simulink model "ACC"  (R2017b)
settings: Solver=FixedStepDiscrete  StartTime=0.0  StopTime=10.0  FixedStep=0.01  RelTol=1e-3  EnableMultiTasking=on
undefined symbols (not defined in the file): ACC_CONST0_NUMB, ACC_CONST1000_NUMB, ACC_CONST100_NUMB, ACC_CONST121_NUMB, ACC_CONST1_NUMB, ACC_CONST2047_NUMB, ACC_CONST60000_NUMB, ACC_CONST60_NUMB, ACC_CONSTF1_NUMB, ACC_RUNTIME_MS, ASWTYPE_FALSE, ASWTYPE_TRUE, CcACC_ACChrgDispSOCPrmt_pct, CcACC_ACChrgMismatch_ms, CcACC_ACChrgPACKVolLim_V, CcACC_ACChrgPACKVolLimTi_ms, CcACC_ACChrgPrmtObcFltLvl_numb, CcACC_ACChrgPrmtVcuFltLvl_numb, CcACC_ACChrgStepCurr_A, CcACC_ACChrgTempPrmtDelayTime_ms, CcACC_ACCrntUnctrolTi_ms, CcACC_ACFullChrgHysVolt_mV, CcACC_ACFullStepChrgTi1_ms, CcACC_ACFullStepChrgTi2_ms, CcACC_ACMaxChrgCurr_A, CcACC_ACStepChrgWaitTime_ms, CcACC_ACStop2DefaultTi_ms, CcACC_ACStop2DefaultTiDelay_ms, CcACC_BatFullResetTime_ms, CcACC_ChrgCrnt0HysVolt_mV, CcACC_ChrgEndDeviationVol1_mV, CcACC_ChrgEndDeviationVol2_mV, CcACC_ChrgEndDeviationVol3_mV, CcACC_ChrgMaxPackVoltLimt_V, CcACC_ChrgPwr1_W, CcACC_ChrgPwr2_W, CcACC_ChrgPwr3_W, CcACC_ChrgSt2StepChrgDeviVol_mV, CcACC_ChrgSt2StepChrgTime_ms, CcACC_ChrgStCutoffTime_ms, CcACC_ChrgStFullChrgCrnt_A, CcACC_CPDutyLowThrhd_pct, CcACC_CrntFilterTi1_cnt, CcACC_CrntFilterTi2_cnt, CcACC_CrntFilterTi2_ms, CcACC_CurrObcPreHeatLowThrhd_A, CcACC_DiffACChrgCrnt_A, CcACC_DiffACChrgCrntTi_ms, CcACC_DispSOCCalStart_pct, CcACC_DispSOCDiff_pct, CcACC_ElecLckRemTimeHold_ms, CcACC_HeatChrgCrnt0Time_ms, CcACC_HeatChrgCrnt1Time_ms, CcACC_Initial500Ti_ms, CcACC_Initial700Ti_ms, CcACC_MaxACChrgCellTemp_C, CcACC_MaxPackVoltLimt_V, CcACC_MinACChrgCellTemp_C, CcACC_MinACChrgCrntRqst_A, CcACC_OBCChrgPwr_W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
libraries: AIWAYS_Powertrain_BMS_lib x94, simulink x2
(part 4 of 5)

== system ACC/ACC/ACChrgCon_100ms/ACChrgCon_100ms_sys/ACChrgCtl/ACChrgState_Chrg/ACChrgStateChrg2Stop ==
  GbACC_ACChrgPrmt_flg : Inport
  GcACC_ACChrgCrntRqst_A : Inport  Port=2
  GcCDP_MaxCellVolt_mV : Inport  Port=3
  GeBTM_HeatReq_enum : Inport  Port=4
  GeVDP_ChrgRqst_enum : Inport  Port=5
  GcUDS_FullChrgCutoffVolt_mV : Inport  Port=6
  GbACC_ACCrntUnctrolFlt_flg : Inport  Port=7
  BMSDebounceStartZero : AIWAYS_Powertrain_BMS_lib/Debounce & Delay/BMSDebounceStartZero
  Constant : Constant  Value=Enum_VDPChrgRqst.Enum_VDPChrgRqst_PowerDown
  Constant1 : Constant  Value=CcACC_ChrgStCutoffTime_ms
  Constant10 : Constant  Value=ACC_RUNTIME_MS
  Constant13 : Constant  Value=ACC_RUNTIME_MS
  Constant3 : Constant  Value=Enum_BTMHeatReq.Enum_BTMHeatReq_Default
  Constant4 : Constant  Value=ASWTYPE_FALSE
  Constant5 : Constant  Value=CcACC_ChrgStFullChrgCrnt_A
  Constant6 : Constant  Value=ASWTYPE_TRUE
  Constant7 : Constant  Value=CcACC_ChrgStCutoffTime_ms
  Data Type Conversion1 : DataTypeConversion
  Data Type Conversion4 : DataTypeConversion
  Logical Operator : Logic  Inputs=3  AllPortsSameDT=off  OutDataTypeStr=boolean
  Logical Operator3 : Logic  Operator=OR  Inputs=4  AllPortsSameDT=off  OutDataTypeStr=boolean
  Relational Operator : RelationalOperator  OutDataTypeStr=boolean
  Relational Operator{1..2,4..5} (4 alike) : RelationalOperator  Operator===  OutDataTypeStr=boolean
  Relational Operator3 : RelationalOperator  Operator=<=  OutDataTypeStr=boolean
  LbACC_ChrgSt2Stop_flg : Outport
  LbACC_FinishInChrgSt_flg : Outport  Port=2
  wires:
  BMSDebounceStartZero/1 -> Logical Operator3/4, LbACC_FinishInChrgSt_flg/1  "LbACC_FinishInChrgSt_flg"
  Logical Operator3/1 -> LbACC_ChrgSt2Stop_flg/1  "LbACC_ChrgSt2Stop_flg"
  Constant4/1 -> Relational Operator2/2
  GbACC_ACChrgPrmt_flg/1 -> Relational Operator2/1
  Constant5/1 -> Relational Operator3/2
  Relational Operator3/1 -> Logical Operator/1
  Logical Operator/1 -> BMSDebounceStartZero/1
  Relational Operator/1 -> Logical Operator/2
  GcACC_ACChrgCrntRqst_A/1 -> Relational Operator3/1
  Constant3/1 -> Relational Operator1/2
  GeBTM_HeatReq_enum/1 -> Data Type Conversion4/1
  Data Type Conversion4/1 -> Relational Operator1/1
  GcCDP_MaxCellVolt_mV/1 -> Relational Operator/1
  Relational Operator1/1 -> Logical Operator/3
  GcUDS_FullChrgCutoffVolt_mV/1 -> Relational Operator/2
  Constant6/1 -> Relational Operator4/2
  GbACC_ACCrntUnctrolFlt_flg/1 -> Relational Operator4/1
  Constant/1 -> Relational Operator5/2
  GeVDP_ChrgRqst_enum/1 -> Data Type Conversion1/1
  Data Type Conversion1/1 -> Relational Operator5/1
  Relational Operator2/1 -> Logical Operator3/1
  Relational Operator4/1 -> Logical Operator3/2
  Relational Operator5/1 -> Logical Operator3/3
  Constant10/1 -> BMSDebounceStartZero/3
  Constant1/1 -> BMSDebounceStartZero/2
  Constant13/1 -> BMSDebounceStartZero/5
  Constant7/1 -> BMSDebounceStartZero/4

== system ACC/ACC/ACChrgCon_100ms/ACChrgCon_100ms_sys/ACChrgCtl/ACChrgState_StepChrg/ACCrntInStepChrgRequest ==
  LbACC_StepChrgVoltReach_flg : Inport  OutDataTypeStr=boolean
  LcACC_StepChrgCrntDec_A : Inport  Port=2
  Constant : Constant  Value=ACC_CONST0_NUMB
  Data Type Conversion2 : DataTypeConversion
  Switch : Switch  Criteria=u2 ~= 0
  LcACC_StepChrgCrntReq_A : Outport
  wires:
  LcACC_StepChrgCrntDec_A/1 -> Switch/3
  Switch/1 -> LcACC_StepChrgCrntReq_A/1  "LcACC_StepChrgCrntReq_A"
  LbACC_StepChrgVoltReach_flg/1 -> Switch/2
  Constant/1 -> Data Type Conversion2/1
  Data Type Conversion2/1 -> Switch/1

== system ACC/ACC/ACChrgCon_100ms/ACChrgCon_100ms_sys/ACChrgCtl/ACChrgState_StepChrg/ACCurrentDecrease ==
  GcACC_ACChrgCrntRqst_A : Inport
  GcUDS_FullChrgCutoffVolt_mV : Inport  Port=2
  GcCDP_MaxCellVolt_mV : Inport  Port=3
  ACStepChrgVoltReach : Subsystem  TreatAsAtomicUnit=on
  BMSDebounceStartZero : AIWAYS_Powertrain_BMS_lib/Debounce & Delay/BMSDebounceStartZero
  Constant1 : Constant  Value=CcACC_StepChrgCutoffTi_ms
  Constant10 : Constant  Value=ACC_RUNTIME_MS
  Constant13 : Constant  Value=ACC_RUNTIME_MS
  Constant4 : Constant  Value=ASWTYPE_FALSE
  Constant5 : Constant  Value=ASWTYPE_FALSE
  Constant6 : Constant  Value=CcACC_StepChrgCutoffTi_ms
  Logical Operator : Logic  Operator=OR  Inputs=3  AllPortsSameDT=off  OutDataTypeStr=boolean
  Relational Operator : RelationalOperator  OutDataTypeStr=boolean
  Subsystem : Subsystem
  Switch : Switch  Criteria=u2 ~= 0  Threshold=""
  Unit Delay : UnitDelay  InitialCondition=ASWTYPE_TRUE  SampleTime=-1  StateName=StateName
  Unit Delay External IC : AIWAYS_Powertrain_BMS_lib/Delay Blocks/Unit Delay External IC
  Unit Delay1 : UnitDelay  InitialCondition=ASWTYPE_FALSE  SampleTime=-1  StateName=StateName
  Unit Delay2 : UnitDelay  InitialCondition=ASWTYPE_FALSE  SampleTime=-1  StateName=StateName
  LbACC_StepChrgVoltReach_flg : Outport
  LcACC_StepChrgCrntDec_A : Outport  Port=2
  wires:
  BMSDebounceStartZero/1 -> Logical Operator/2
  Unit Delay/1 -> Subsystem/Enable, Logical Operator/3
  Switch/1 -> Logical Operator/1
  Unit Delay2/1 -> Switch/3
  Constant5/1 -> Switch/1
  Unit Delay1/1 -> Switch/2
  Logical Operator/1 -> LbACC_StepChrgVoltReach_flg/1, ACStepChrgVoltReach/Enable, Unit Delay2/1  "LbACC_StepChrgVoltReach_flg"
  Constant4/1 -> Unit Delay/1
  Relational Operator/1 -> BMSDebounceStartZero/1
  GcCDP_MaxCellVolt_mV/1 -> Relational Operator/1
  GcUDS_FullChrgCutoffVolt_mV/1 -> Relational Operator/2
  ACStepChrgVoltReach/1(LbACC_ACStepWaitReach_flg) -> Unit Delay1/1
  Unit Delay External IC/1 -> ACStepChrgVoltReach/1(LcACC_LastCrntRqst_A)  "LcACC_LastCrntRqst_A"
  GcACC_ACChrgCrntRqst_A/1 -> Subsystem/1(GcACC_ACChrgCrntRqst_A)
  ACStepChrgVoltReach/2(LcACC_StepChrgCrntDec_A) -> LcACC_StepChrgCrntDec_A/1, Unit Delay External IC/1
  Constant6/1 -> BMSDebounceStartZero/4
  Constant10/1 -> BMSDebounceStartZero/3
  Constant13/1 -> BMSDebounceStartZero/5
  Constant1/1 -> BMSDebounceStartZero/2
  Subsystem/1(LcACC_LockACChrgCrntRqst_A) -> Unit Delay External IC/2

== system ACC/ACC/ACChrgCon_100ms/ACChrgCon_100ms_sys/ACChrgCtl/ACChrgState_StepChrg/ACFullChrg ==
  LcACC_StepChrgCrntReq_A : Inport
  GcCDP_MaxCellVolt_mV : Inport  Port=2
  GcUDS_FullChrgCutoffVolt_mV : Inport  Port=3
  Add : Sum
  BMSDebounceStartZero : AIWAYS_Powertrain_BMS_lib/Debounce & Delay/BMSDebounceStartZero
  BMSDebounceStartZero1 : AIWAYS_Powertrain_BMS_lib/Debounce & Delay/BMSDebounceStartZero
  Constant : Constant  Value=CcACC_StepChrgFullChrgCrnt_A
  Constant1 : Constant  Value=CcACC_ACFullStepChrgTi1_ms
  Constant{9..11,13} (4 alike) : Constant  Value=ACC_RUNTIME_MS
  Constant2 : Constant  Value=CcACC_ACFullStepChrgTi2_ms
  Constant3 : Constant  Value=CcACC_ACFullChrgHysVolt_mV
  Constant7 : Constant  Value=CcACC_ACFullStepChrgTi2_ms
  Constant8 : Constant  Value=CcACC_ACFullStepChrgTi1_ms
  Logical Operator1 : Logic  Operator=OR  AllPortsSameDT=off  OutDataTypeStr=boolean
  Logical Operator2 : Logic  AllPortsSameDT=off  OutDataTypeStr=boolean
  Relational Operator : RelationalOperator  Operator=<=  OutDataTypeStr=boolean
  Relational Operator1 : RelationalOperator  OutDataTypeStr=boolean
  Relational Operator2 : RelationalOperator  OutDataTypeStr=boolean
  LbACC_FinishInStepChrg_flg : Outport
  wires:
  LcACC_StepChrgCrntReq_A/1 -> Relational Operator/1
  Relational Operator1/1 -> BMSDebounceStartZero/1
  GcCDP_MaxCellVolt_mV/1 -> Relational Operator2/1, Relational Operator1/1
  GcUDS_FullChrgCutoffVolt_mV/1 -> Add/1, Relational Operator2/2
  Add/1 -> Relational Operator1/2
  Constant3/1 -> Add/2
  BMSDebounceStartZero/1 -> Logical Operator1/2
  Logical Operator1/1 -> LbACC_FinishInStepChrg_flg/1  "LbACC_FinishInStepChrg_flg"
  Constant/1 -> Relational Operator/2
  Relational Operator/1 -> Logical Operator2/1
  Relational Operator2/1 -> Logical Operator2/2
  Logical Operator2/1 -> BMSDebounceStartZero1/1
  BMSDebounceStartZero1/1 -> Logical Operator1/1
  Constant8/1 -> BMSDebounceStartZero/4
  Constant10/1 -> BMSDebounceStartZero/3
  Constant13/1 -> BMSDebounceStartZero/5
  Constant1/1 -> BMSDebounceStartZero/2
  Constant7/1 -> BMSDebounceStartZero1/2
  Constant11/1 -> BMSDebounceStartZero1/5
  Constant9/1 -> BMSDebounceStartZero1/3
  Constant2/1 -> BMSDebounceStartZero1/4

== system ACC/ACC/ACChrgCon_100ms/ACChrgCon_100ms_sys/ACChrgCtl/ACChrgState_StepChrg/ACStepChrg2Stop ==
  LbACC_FinishInStepChrg_flg : Inport
  GbACC_ACChrgPrmt_flg : Inport  Port=2
  GeVDP_ChrgRqst_enum : Inport  Port=3
  Constant : Constant  Value=Enum_VDPChrgRqst.Enum_VDPChrgRqst_PowerDown
  Constant3 : Constant  Value=ASWTYPE_FALSE
  Data Type Conversion1 : DataTypeConversion
  Logical Operator1 : Logic  Operator=OR  Inputs=3  AllPortsSameDT=off  OutDataTypeStr=boolean
  Relational Operator1 : RelationalOperator  Operator===  OutDataTypeStr=boolean
  Relational Operator5 : RelationalOperator  Operator===  OutDataTypeStr=boolean
  LbACC_StepChrg2Stop_flg : Outport
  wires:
  GbACC_ACChrgPrmt_flg/1 -> Relational Operator1/1
  Logical Operator1/1 -> LbACC_StepChrg2Stop_flg/1  "LbACC_StepChrg2Stop_flg"
  Relational Operator1/1 -> Logical Operator1/1
  Constant3/1 -> Relational Operator1/2
  LbACC_FinishInStepChrg_flg/1 -> Logical Operator1/2
  GeVDP_ChrgRqst_enum/1 -> Data Type Conversion1/1
  Constant/1 -> Relational Operator5/2
  Data Type Conversion1/1 -> Relational Operator5/1
  Relational Operator5/1 -> Logical Operator1/3

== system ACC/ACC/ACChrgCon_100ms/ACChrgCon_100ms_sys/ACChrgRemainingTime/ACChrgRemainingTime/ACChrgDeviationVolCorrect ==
  GcODP_MaxPwrObcChrg_W : Inport
  Constant13 : Constant  Value=CcACC_ChrgEndDeviationVol3_mV
  Constant15 : Constant  Value=CcACC_ChrgPwr1_W
  Constant16 : Constant  Value=CcACC_ChrgEndDeviationVol1_mV
  Constant17 : Constant  Value=CcACC_ChrgPwr2_W
  Constant18 : Constant  Value=CcACC_ChrgEndDeviationVol2_mV
  Constant19 : Constant  Value=CcACC_ChrgPwr1_W
  Data Type Conversion1 : DataTypeConversion
  Logical Operator1 : Logic  AllPortsSameDT=off  OutDataTypeStr=boolean
  Relational Operator2 : RelationalOperator  OutDataTypeStr=boolean
  Relational Operator3 : RelationalOperator  Operator=<=  OutDataTypeStr=boolean
  Relational Operator4 : RelationalOperator  Operator=>  OutDataTypeStr=boolean
  Switch5 : Switch  Criteria=u2 ~= 0
  Switch6 : Switch  Criteria=u2 ~= 0
  LcACC_ChrgEndDeviationVol_mV : Outport
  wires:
  Relational Operator4/1 -> Switch5/2
  Constant16/1 -> Switch5/1
  Constant15/1 -> Relational Operator4/2
  Constant17/1 -> Relational Operator2/2
  Constant13/1 -> Switch6/3
  Data Type Conversion1/1 -> Relational Operator3/1, Relational Operator2/1, Relational Operator4/1
  Relational Operator2/1 -> Logical Operator1/1
  Constant18/1 -> Switch6/1
  Switch6/1 -> Switch5/3
  Constant19/1 -> Relational Operator3/2
  GcODP_MaxPwrObcChrg_W/1 -> Data Type Conversion1/1
  Relational Operator3/1 -> Logical Operator1/2
  Switch5/1 -> LcACC_ChrgEndDeviationVol_mV/1
  Logical Operator1/1 -> Switch6/2

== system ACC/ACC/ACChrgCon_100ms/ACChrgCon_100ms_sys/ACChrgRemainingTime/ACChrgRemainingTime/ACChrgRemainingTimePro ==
  LcACC_TiRemCalc_min : Inport
  GeODP_ObcElecLck_enum : Inport  Port=2
  ACChrgRemainingTimeChange : Subsystem
  ACChrgRemainingTimeEleclckPro : Subsystem
  BMSDelay : AIWAYS_Powertrain_BMS_lib/Debounce & Delay/BMSDelay
  Bus Creator1 : BusCreator  Inputs=3
  Bus Selector1 : BusSelector  OutputSignals=LcACC_ChrgingTiRem_min
  Bus Selector2 : BusSelector  OutputSignals=LcACC_ChrgingTiRem_min,signal3
  Bus Selector3 : BusSelector  OutputSignals=signal3
  Bus Selector4 : BusSelector  OutputSignals=LcACC_TiRemCalcRound_min
  Bus Selector5 : BusSelector  OutputSignals=LcACC_ChrgingTiRem_min,LcACC_TiRemCalcRound_min
  Constant : Constant  Value=ASWTYPE_TRUE
  Constant1 : Constant  Value=CcACC_RemTimeChangeStep_min
  Constant2 : Constant  Value=CcACC_RemTimeStepChange_min
  Constant3 : Constant  Value=CcACC_RemTimeStepChange_min
  Constant4 : Constant  Value=CcACC_Initial500Ti_ms
  Constant5 : Constant  Value=ACC_RUNTIME_MS
  Data Type Conversion1 : DataTypeConversion  OutDataTypeStr=uint16
  Product1 : Product  Inputs=*/  OutDataTypeStr=int16
  Product5 : Product  OutDataTypeStr=Inherit: Inherit via back propagation
  Relational Operator1 : RelationalOperator  OutDataTypeStr=boolean
  Relational Operator2 : RelationalOperator  Operator===  OutDataTypeStr=boolean
  Relational Operator3 : RelationalOperator  Operator=<  OutDataTypeStr=boolean
  Relational Operator4 : RelationalOperator  OutDataTypeStr=boolean
  StateRetention : Subsystem
  Switch{1..5} (5 alike) : Switch  Criteria=u2 ~= 0
  Unit Delay : UnitDelay  SampleTime=-1  StateName=StateName
  LcACC_ChrgingTiRem_min : Outport
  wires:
  LcACC_TiRemCalc_min/1 -> Data Type Conversion1/1
  Constant1/1 -> Product5/2, Product1/2
  Product1/1 -> Product5/1
  Constant2/1 -> Relational Operator1/2
  Relational Operator1/1 -> Switch1/2
  Bus Selector5/2 -> ACChrgRemainingTimeChange/1(LcACC_TiRemCalcRound_min), Relational Operator2/2  "<LcACC_TiRemCalcRound_min>"
  Relational Operator2/1 -> StateRetention/1(set)
  StateRetention/1(LcACC_TiRemEq_flg) -> Switch2/2
  ACChrgRemainingTimeChange/1(LcACC_TiRemChanged_flg) -> Switch2/3
  Constant4/1 -> BMSDelay/3
  Constant5/1 -> BMSDelay/2
  Constant/1 -> BMSDelay/1
  BMSDelay/1 -> Switch3/2
  ACChrgRemainingTimeEleclckPro/1(LcACC_TiRemEleclckPro_min) -> Switch3/1
  Switch2/1 -> Switch1/1
  Switch5/1 -> Bus Creator1/2  "LcACC_TiRemCalcRound_min"
  Bus Selector5/1 -> Switch2/1, Relational Operator2/1  "<LcACC_ChrgingTiRem_min>"
  Unit Delay/1 -> Bus Creator1/1, ACChrgRemainingTimeEleclckPro/1(LcACC_ChrgingTiRem_min)  "LcACC_ChrgingTiRem_min"
  Bus Selector1/1 -> ACChrgRemainingTimeChange/2(LcACC_ChrgingTiRem_min)  "<LcACC_ChrgingTiRem_min>"
  Relational Operator3/1 -> Switch4/2
  Bus Selector3/1 -> Relational Operator1/1  "<signal3>"
  Bus Selector2/1 -> Relational Operator3/1, Switch4/1  "<LcACC_ChrgingTiRem_min>"
  Bus Creator1/1 -> Bus Selector3/1, Bus Selector4/1, Bus Selector2/1, Bus Selector1/1, Bus Selector5/1
  Bus Selector2/2 -> Switch4/3, Relational Operator3/2  "<signal3>"
  Switch4/1 -> Switch1/3
  Bus Selector4/1 -> Switch3/3  "<LcACC_TiRemCalcRound_min>"
  Switch1/1 -> ACChrgRemainingTimeEleclckPro/3(LcACC_TiRemPro_min)
  GeODP_ObcElecLck_enum/1 -> ACChrgRemainingTimeEleclckPro/2(GeODP_ObcElecLck_enum)
  Data Type Conversion1/1 -> Product1/1, Relational Operator4/1, Switch5/3, Bus Creator1/3
  Constant3/1 -> Relational Operator4/2
  Relational Operator4/1 -> Switch5/2
  Product5/1 -> Switch5/1
  Switch3/1 -> LcACC_ChrgingTiRem_min/1, Unit Delay/1

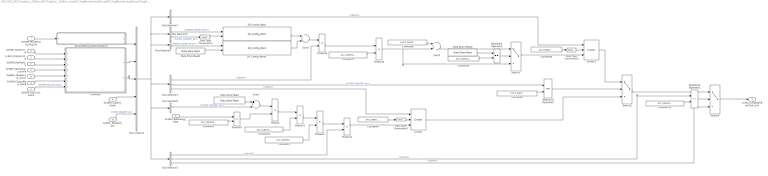
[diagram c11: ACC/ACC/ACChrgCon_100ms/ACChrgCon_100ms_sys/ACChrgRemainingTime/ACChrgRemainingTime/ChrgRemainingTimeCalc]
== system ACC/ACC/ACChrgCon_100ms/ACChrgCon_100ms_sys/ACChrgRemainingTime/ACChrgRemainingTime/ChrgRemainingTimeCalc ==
  GcHDP_PackCrnt_A : Inport
  LcACC_FilterCrnt1_A : Inport  Port=2
  GcHDP_PackVolt_V : Inport  Port=3
  GeODP_ObcCcSt_enum : Inport  Port=4
  GcODP_ObcCpDuty_numb : Inport  Port=5
  GcVDP_ChrgLdReq_numb : Inport  Port=6
  GcODP_MaxPwrObcChrg_W : Inport  Port=7
  GcUDS_BatEnergy_kWh : Inport  Port=8
  GeUDS_CapSel_enum : Inport  Port=9
  GcSOC_DispSOC_pct : Inport  Port=10
  GeODP_ObcElecLck_enum : Inport  Port=11
  2D_Config_Word : AIWAYS_Powertrain_BMS_lib/Signals/2D_Config_Word  Default_Cal_Breakpoint1_Name=CaACC_RemCapDispSOCTable_pct  Default_Cal_Table1_Name=CaACC_CATL177RemCapTable_Wh  CATL153Ah_Cal_Breakpoint1_Name=CaACC_RemCapDispSOCTable_pct  CATL153Ah_Cal_Table1_Name=CaACC_CATL177RemCapTable_Wh  CATL180Ah_Cal_Breakpoint1_Name=CaACC_RemCapDispSOCTable_pct  CATL180Ah_Cal_Table1_Name=CaACC_CATL177RemCapTable_Wh  CATL177Ah_Cal_Breakpoint1_Name=CaACC_RemCapDispSOCTable_pct  CATL177Ah_Cal_Table1_Name=CaACC_CATL177RemCapTable_Wh  CATL203Ah_Cal_Breakpoint1_Name=CaACC_RemCapDispSOCTable_pct  CATL203Ah_Cal_Table1_Name=CaACC_CATL203RemCapTable_Wh  CATL51Ah_Cal_Breakpoint1_Name=CaACC_RemCapDispSOCTable_pct  CATL51Ah_Cal_Table1_Name=CaACC_CATL177RemCapTable_Wh  CATL132Ah_Cal_Breakpoint1_Name=CaACC_RemCapDispSOCTable_pct  CATL132Ah_Cal_Table1_Name=CaACC_CATL177RemCapTable_Wh  XWD75Ah_Cal_Breakpoint1_Name=CaACC_RemCapDispSOCTable_pct  XWD75Ah_Cal_Table1_Name=CaACC_XWD75RemCapTable_Wh  TFE177Ah_Cal_Breakpoint1_Name=CaACC_RemCapDispSOCTable_pct  TFE177Ah_Cal_Table1_Name=CaACC_CATL177RemCapTable_Wh  CATLCTP248Ah_Cal_Breakpoint1_Name=CaACC_RemCapDispSOCTable_pct  CATLCTP248Ah_Cal_Table1_Name=CaACC_CATL177RemCapTable_Wh
  2D_Config_Word1 : AIWAYS_Powertrain_BMS_lib/Signals/2D_Config_Word  Default_Cal_Breakpoint1_Name=CaACC_RemCapDispSOCTable_pct  Default_Cal_Table1_Name=CaACC_CATL177RemCapTable_Wh  CATL153Ah_Cal_Breakpoint1_Name=CaACC_RemCapDispSOCTable_pct  CATL153Ah_Cal_Table1_Name=CaACC_CATL177RemCapTable_Wh  CATL180Ah_Cal_Breakpoint1_Name=CaACC_RemCapDispSOCTable_pct  CATL180Ah_Cal_Table1_Name=CaACC_CATL177RemCapTable_Wh  CATL177Ah_Cal_Breakpoint1_Name=CaACC_RemCapDispSOCTable_pct  CATL177Ah_Cal_Table1_Name=CaACC_CATL177RemCapTable_Wh  CATL203Ah_Cal_Breakpoint1_Name=CaACC_RemCapDispSOCTable_pct  CATL203Ah_Cal_Table1_Name=CaACC_CATL203RemCapTable_Wh  CATL51Ah_Cal_Breakpoint1_Name=CaACC_RemCapDispSOCTable_pct  CATL51Ah_Cal_Table1_Name=CaACC_CATL177RemCapTable_Wh  CATL132Ah_Cal_Breakpoint1_Name=CaACC_RemCapDispSOCTable_pct  CATL132Ah_Cal_Table1_Name=CaACC_CATL177RemCapTable_Wh  XWD75Ah_Cal_Breakpoint1_Name=CaACC_RemCapDispSOCTable_pct  XWD75Ah_Cal_Table1_Name=CaACC_XWD75RemCapTable_Wh  TFE177Ah_Cal_Breakpoint1_Name=CaACC_RemCapDispSOCTable_pct  TFE177Ah_Cal_Table1_Name=CaACC_CATL177RemCapTable_Wh  CATLCTP248Ah_Cal_Breakpoint1_Name=CaACC_RemCapDispSOCTable_pct  CATLCTP248Ah_Cal_Table1_Name=CaACC_CATL177RemCapTable_Wh
  ACChrgRemainingTimeUpLmt : Subsystem
  Bus Creator1 : BusCreator  Inputs=5
  Bus Selector1 : BusSelector  OutputSignals=signal1
  Bus Selector2 : BusSelector  OutputSignals=signal2,signal3,signal1
  Bus Selector3 : BusSelector  OutputSignals=signal2,GcSOC_DispSOC_pct,signal1
  Bus Selector4 : BusSelector  OutputSignals=GeUDS_CapSel_enum
  Bus Selector5 : BusSelector  OutputSignals=GeUDS_CapSel_enum,GcSOC_DispSOC_pct
  Bus Selector6 : BusSelector  OutputSignals=GcSOC_DispSOC_pct
  Constant1 : Constant  Value=ACC_CONST1000_NUMB
  Constant12 : Constant  Value=ACC_CONSTF1_NUMB
  Constant2 : Constant  Value=ACC_CONST100_NUMB
  Constant3 : Constant  Value=ACC_CONST60_NUMB
  Constant4 : Constant  Value=ACC_CONST1_NUMB
  Constant5 : Constant  Value=CcACC_DispSOCCalStart_pct
  Constant6 : Constant  Value=CcACC_SOC99ToEndRemTi_min
  Constant7 : Constant  Value=ACC_CONST60_NUMB
  Constant8 : Constant  Value=ACC_CONST1_NUMB
  Constant9 : Constant  Value=ACC_CONST100_NUMB
  CrntFilter : Subsystem
  Data Store Read : AIWAYS_Powertrain_BMS_lib/Signals/Data Store Read  Priority=0  DSR=EcNVM_ChrgPermitMaxSOC_pct
  Data Store Read1 : AIWAYS_Powertrain_BMS_lib/Signals/Data Store Read  Priority=0  DSR=EcNVM_ChrgPermitMaxSOC_pct
  Data Store Read2 : AIWAYS_Powertrain_BMS_lib/Signals/Data Store Read  Priority=0  DSR=EcNVM_ChrgPermitMaxSOC_pct
  Data Type Conversion1 : DataTypeConversion
  Data Type Conversion2 : DataTypeConversion
  Data Type Conversion3 : DataTypeConversion  RndMeth=Round
  Limiter : AIWAYS_Powertrain_BMS_lib/Nonlinear Blocks/Limiter
  Limiter1 : AIWAYS_Powertrain_BMS_lib/Nonlinear Blocks/Limiter
  Product{,2,4..5} (4 alike) : Product  OutDataTypeStr=Inherit: Inherit via back propagation
  Product1 : Product  Inputs=*/  OutDataTypeStr=Inherit: Inherit via back propagation
  Product3 : Product  Inputs=*/  OutDataTypeStr=Inherit: Inherit via back propagation
  Product6 : Product  Inputs=*/  OutDataTypeStr=Inherit: Inherit via back propagation
  Relational Operator1 : RelationalOperator  Operator=<=  OutDataTypeStr=boolean
  Relational Operator2 : RelationalOperator  OutDataTypeStr=boolean
  Relational Operator3 : RelationalOperator  Operator===  OutDataTypeStr=boolean
  Sum1 : Sum  Inputs=+-  OutDataTypeStr=Inherit: Inherit via back propagation  RndMeth=Zero
  Sum2 : Sum  Inputs=+-  OutDataTypeStr=Inherit: Inherit via back propagation  RndMeth=Zero
  Sum3 : Sum  OutDataTypeStr=Inherit: Inherit via back propagation  RndMeth=Zero
  Switch1 : Switch  Criteria=u2 ~= 0
  Switch2 : Switch  Criteria=u2 ~= 0
  Switch4 : Switch  Criteria=u2 ~= 0
  LcACC_ChrgingTiRemCalc_min : Outport
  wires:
  Data Store Read/1 -> Sum1/1
  GcSOC_DispSOC_pct/1 -> Bus Creator1/5  "GcSOC_DispSOC_pct"
  Sum1/1 -> Product/1
  Product4/1 -> Product/2
  Product/1 -> Product1/1
  Constant2/1 -> Product1/2
  Product1/1 -> Product2/1
  Constant3/1 -> Product2/2
  Product2/1 -> Product3/1
  Constant12/1 -> Relational Operator1/2
  Relational Operator1/1 -> Switch4/2
  Product3/1 -> Limiter/3
  Switch4/1 -> LcACC_ChrgingTiRemCalc_min/1
  GeODP_ObcCcSt_enum/1 -> CrntFilter/7(GeODP_ObcCcSt_enum)  "GeODP_ObcCcSt_enum"
  Constant6/1 -> Sum3/1
  Product5/1 -> Switch1/3, Sum3/2
  Constant7/1 -> Product5/2
  Product6/1 -> Product5/1
  Limiter/1 -> Switch2/3
  Switch1/1 -> Limiter1/3
  Relational Operator2/1 -> Switch2/2
  Switch2/1 -> Switch4/1
  Data Type Conversion2/1 -> Limiter1/2
  Limiter1/1 -> Switch2/1
  Bus Selector2/1 -> Product3/2  "<signal2>"
  GcHDP_PackCrnt_A/1 -> CrntFilter/1(GcHDP_PackCrnt_A)
  LcACC_FilterCrnt1_A/1 -> CrntFilter/2(LcACC_FilterCrnt1_A)
  GcHDP_PackVolt_V/1 -> CrntFilter/3(GcHDP_PackVolt_V)
  Bus Selector2/2 -> Relational Operator1/1  "<signal3>"
  Bus Selector3/3 -> Limiter/1  "<signal1>"
  CrntFilter/1(LcACC_FilterPwr_W) -> Bus Creator1/2
  CrntFilter/2(LcACC_FilterCrnt_A) -> Bus Creator1/3
  ACChrgRemainingTimeUpLmt/1(LcACC_RemainingTimeUpLmt_min) -> Bus Creator1/1
  Bus Creator1/1 -> Bus Selector2/1, Bus Selector6/1, Bus Selector3/1, Bus Selector1/1, Bus Selector5/1, Bus Selector4/1
  Bus Selector1/1 -> Limiter1/1  "<signal1>"
  Bus Selector3/1 -> Product6/2  "<signal2>"
  Bus Selector2/3 -> Switch4/3  "<signal1>"
  Bus Selector5/2 -> Data Type Conversion3/1  "<GcSOC_DispSOC_pct>"
  GcODP_ObcCpDuty_numb/1 -> CrntFilter/4(GcODP_ObcCpDuty_numb)
  GeODP_ObcElecLck_enum/1 -> CrntFilter/5(GeODP_ObcElecLck_enum)
  GcVDP_ChrgLdReq_numb/1 -> CrntFilter/6(GcVDP_ChrgLdReq_numb)
  GcODP_MaxPwrObcChrg_W/1 -> ACChrgRemainingTimeUpLmt/1(GcODP_MaxPwrObcChrg_W)
  GcUDS_BatEnergy_kWh/1 -> Product4/1
  Constant1/1 -> Product4/2
  GeUDS_CapSel_enum/1 -> Bus Creator1/4
  2D_Config_Word/1 -> Sum2/1
  Bus Selector5/1 -> 2D_Config_Word/1  "<GeUDS_CapSel_enum>"
  Constant4/1 -> Data Type Conversion1/1
  Data Type Conversion1/1 -> Limiter/2
  Bus Selector6/1 -> Sum1/2  "<GcSOC_DispSOC_pct>"
  Bus Selector3/2 -> Relational Operator2/1  "<GcSOC_DispSOC_pct>"
  Constant5/1 -> Relational Operator2/2
  Bus Selector4/1 -> 2D_Config_Word1/1  "<GeUDS_CapSel_enum>"
  2D_Config_Word1/1 -> Sum2/2
  Sum2/1 -> Product6/1
  Constant8/1 -> Data Type Conversion2/1
  Data Store Read2/1 -> Relational Operator3/1
  Constant9/1 -> Relational Operator3/2
  Relational Operator3/1 -> Switch1/2
  Sum3/1 -> Switch1/1
  Data Store Read1/1 -> 2D_Config_Word1/2
  Data Type Conversion3/1 -> 2D_Config_Word/2

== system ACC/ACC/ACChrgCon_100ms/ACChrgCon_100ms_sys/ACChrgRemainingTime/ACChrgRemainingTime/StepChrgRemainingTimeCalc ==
  Enable : EnablePort  StatesWhenEnabling=reset
  Constant1 : Constant  Value=ACC_CONST60000_NUMB
  Constant2 : Constant  Value=ACC_CONST1_NUMB
  Constant3 : Constant  Value=ACC_RUNTIME_MS
  Constant4 : Constant  Value=CcACC_SOC99ToEndRemTi_min
  Data Type Conversion2 : DataTypeConversion
  Limiter : AIWAYS_Powertrain_BMS_lib/Nonlinear Blocks/Limiter
  Product1 : Product  Inputs=*/  OutDataTypeStr=Inherit: Inherit via back propagation
  Sum1 : Sum  Inputs=+-  OutDataTypeStr=Inherit: Inherit via back propagation  RndMeth=Zero
  Unit Delay : UnitDelay  InitialCondition=CcACC_SOC99ToEndRemTi_min  SampleTime=-1  StateName=StateName
  LcACC_StepChrgTiRemCalc_min : Outport
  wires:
  Constant3/1 -> Product1/1
  Constant1/1 -> Product1/2
  Product1/1 -> Sum1/2
  Sum1/1 -> Unit Delay/1, Limiter/3
  Unit Delay/1 -> Sum1/1
  Limiter/1 -> LcACC_StepChrgTiRemCalc_min/1
  Constant2/1 -> Data Type Conversion2/1
  Constant4/1 -> Limiter/1
  Data Type Conversion2/1 -> Limiter/2

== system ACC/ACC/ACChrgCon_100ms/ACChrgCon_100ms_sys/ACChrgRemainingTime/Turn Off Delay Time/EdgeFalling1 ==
  note: Edge Falling
  u : Inport  OutDataTypeStr=boolean
  AND : Logic  OutDataTypeStr=boolean
  OR1 : Logic  Operator=NOT  OutDataTypeStr=boolean
  Unit Delay : UnitDelay  SampleTime=-1
  y : Outport  OutDataTypeStr=boolean
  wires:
  u/1 -> Unit Delay/1, OR1/1
  AND/1 -> y/1
  Unit Delay/1 -> AND/2
  OR1/1 -> AND/1

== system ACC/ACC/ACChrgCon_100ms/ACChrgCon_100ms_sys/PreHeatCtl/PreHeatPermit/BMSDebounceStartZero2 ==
  Signal : Inport
  Hearl2Fault : Inport  Port=2
  FaultStep : Inport  Port=3
  Fault2Heal : Inport  Port=4
  HealStep : Inport  Port=5
  Compare To Zero : simulink/Logic and Bit Operations/Compare To Zero  relop===  OutDataTypeStr=boolean
  FaultProcess : Subsystem
  HealProcess : Subsystem
  Switch : Switch  Criteria=u2 ~= 0
  Unit Delay : UnitDelay  SampleTime=-1  StateName=StateName
  FaultFlag : Outport  OutDataTypeStr=boolean
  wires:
  Compare To Zero/1 -> Switch/2
  Unit Delay/1 -> Compare To Zero/1, FaultProcess/4(FaultFlagOldState), HealProcess/4(FaultFlagOldState)
  HealStep/1 -> HealProcess/3(HealStep)
  Fault2Heal/1 -> HealProcess/2(Fault2Heal)
  Signal/1 -> FaultProcess/1(Signal), HealProcess/1(Signal)
  FaultStep/1 -> FaultProcess/3(FaultStep)
  Hearl2Fault/1 -> FaultProcess/2(Hearl2Fault)
  Switch/1 -> Unit Delay/1, FaultFlag/1
  HealProcess/1(FaultFlag) -> Switch/3
  FaultProcess/1(FaultFlag) -> Switch/1

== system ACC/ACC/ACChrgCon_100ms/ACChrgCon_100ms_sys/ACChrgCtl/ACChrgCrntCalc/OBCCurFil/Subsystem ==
  set : Inport
  clear : Inport  Port=2
  Logical Operator1 : Logic  AllPortsSameDT=off  OutDataTypeStr=boolean
  Logical Operator2 : Logic  Operator=OR  AllPortsSameDT=off  OutDataTypeStr=boolean
  Logical2 : Logic  Operator=NOT  OutDataTypeStr=boolean
  Unit Delay1 : UnitDelay  SampleTime=-1  StateName=StateName
  Q : Outport
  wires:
  set/1 -> Logical Operator2/2
  Logical Operator1/1 -> Q/1, Unit Delay1/1
  Logical Operator2/1 -> Logical Operator1/1
  clear/1 -> Logical2/1
  Unit Delay1/1 -> Logical Operator2/1
  Logical2/1 -> Logical Operator1/2

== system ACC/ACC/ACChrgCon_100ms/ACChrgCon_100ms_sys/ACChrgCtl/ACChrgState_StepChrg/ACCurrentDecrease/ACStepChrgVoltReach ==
  LcACC_LastCrntRqst_A : Inport
  Enable : EnablePort  StatesWhenEnabling=reset
  Add : Sum  Inputs=+-  AccumDataTypeStr=single  OutDataTypeStr=single
  BMSDelay : AIWAYS_Powertrain_BMS_lib/Debounce & Delay/BMSDelay
  Constant : Constant  Value=ASWTYPE_TRUE
  Constant2 : Constant  Value=ACC_RUNTIME_MS
  Constant3 : Constant  Value=CcACC_ACChrgStepCurr_A
  Constant4 : Constant  Value=ACC_CONST0_NUMB
  Constant5 : Constant  Value=CcACC_ACStepChrgWaitTime_ms
  Data Type Conversion2 : DataTypeConversion
  Limiter : AIWAYS_Powertrain_BMS_lib/Nonlinear Blocks/Limiter
  Switch : Switch  Criteria=u2 ~= 0
  LbACC_ACStepWaitReach_flg : Outport
  LcACC_StepChrgCrntDec_A : Outport  Port=2
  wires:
  BMSDelay/1 -> Switch/2, LbACC_ACStepWaitReach_flg/1  "LbACC_ACStepWaitReach_flg"
  LcACC_LastCrntRqst_A/1 -> Limiter/1, Add/1, Switch/3
  Constant3/1 -> Add/2
  Add/1 -> Limiter/3
  Limiter/1 -> Switch/1
  Constant/1 -> BMSDelay/1
  Constant2/1 -> BMSDelay/2
  Constant5/1 -> BMSDelay/3
  Switch/1 -> LcACC_StepChrgCrntDec_A/1  "LcACC_StepChrgCrntDec_A"
  Constant4/1 -> Data Type Conversion2/1
  Data Type Conversion2/1 -> Limiter/2

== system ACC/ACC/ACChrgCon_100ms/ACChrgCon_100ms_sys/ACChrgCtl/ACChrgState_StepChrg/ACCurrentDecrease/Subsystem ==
  GcACC_ACChrgCrntRqst_A : Inport
  Enable : EnablePort  StatesWhenEnabling=reset
  Signal Conversion : SignalConversion  ConversionOutput=Contiguous copy  OverrideOpt=off
  LcACC_LockACChrgCrntRqst_A : Outport
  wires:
  GcACC_ACChrgCrntRqst_A/1 -> Signal Conversion/1
  Signal Conversion/1 -> LcACC_LockACChrgCrntRqst_A/1  "LcACC_LockACChrgCrntRqst_A"

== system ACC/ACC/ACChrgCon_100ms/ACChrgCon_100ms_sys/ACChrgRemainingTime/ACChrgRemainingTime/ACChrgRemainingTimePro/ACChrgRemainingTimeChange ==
  LcACC_TiRemCalcRound_min : Inport
  LcACC_ChrgingTiRem_min : Inport  Port=2
  BMSDelay : AIWAYS_Powertrain_BMS_lib/Debounce & Delay/BMSDelay
  BMSDelay1 : AIWAYS_Powertrain_BMS_lib/Debounce & Delay/BMSDelay
  Bus Creator1 : BusCreator  Inputs=2
  Bus Selector1 : BusSelector  OutputSignals=LcACC_ChrgingTiRem_min
  Bus Selector5 : BusSelector  OutputSignals=LcACC_TiRemCalcRound_min,LcACC_ChrgingTiRem_min
  Bus Selector6 : BusSelector  OutputSignals=LcACC_TiRemCalcRound_min,LcACC_ChrgingTiRem_min
  Constant1 : Constant  Value=CcACC_RemTimeChangeStep_min
  Constant2 : Constant  Value=CcACC_RemTimeChangePrmtDelayTi_ms
  Constant3 : Constant  Value=CcACC_RemTimeChangePrmtDelayTi_ms
  Constant4 : Constant  Value=ACC_RUNTIME_MS
  Constant5 : Constant  Value=ACC_RUNTIME_MS
  Constant6 : Constant  Value=CcACC_RemTimeChangeStep_min
  Relational Operator3 : RelationalOperator  Operator=>  OutDataTypeStr=boolean
  Relational Operator4 : RelationalOperator  Operator=<  OutDataTypeStr=boolean
  Sum1 : Sum  Inputs=+-  OutDataTypeStr=Inherit: Inherit via back propagation  RndMeth=Zero
  Sum2 : Sum  OutDataTypeStr=Inherit: Inherit via back propagation  RndMeth=Zero
  Switch3 : Switch  Criteria=u2 ~= 0
  Switch4 : Switch  Criteria=u2 ~= 0
  LcACC_TiRemChanged_flg : Outport
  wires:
  Sum2/1 -> Switch3/1
  Constant1/1 -> Sum2/1
  BMSDelay/1 -> Switch3/2
  Constant5/1 -> BMSDelay/2
  Constant2/1 -> BMSDelay/3
  Constant4/1 -> BMSDelay1/2
  BMSDelay1/1 -> Switch4/2
  Constant6/1 -> Sum1/2
  Sum1/1 -> Switch4/1
  Switch4/1 -> Switch3/3
  LcACC_TiRemCalcRound_min/1 -> Bus Creator1/1
  LcACC_ChrgingTiRem_min/1 -> Bus Creator1/2
  Bus Creator1/1 -> Bus Selector6/1, Bus Selector5/1, Bus Selector1/1
  Bus Selector1/1 -> Sum2/2  "<LcACC_ChrgingTiRem_min>"
  Bus Selector5/2 -> Sum1/1, Relational Operator3/2  "<LcACC_ChrgingTiRem_min>"
  Bus Selector5/1 -> Relational Operator3/1  "<LcACC_TiRemCalcRound_min>"
  Relational Operator3/1 -> BMSDelay/1
  Bus Selector6/1 -> Relational Operator4/1  "<LcACC_TiRemCalcRound_min>"
  Relational Operator4/1 -> BMSDelay1/1
  Constant3/1 -> BMSDelay1/3
  Bus Selector6/2 -> Switch4/3, Relational Operator4/2  "<LcACC_ChrgingTiRem_min>"
  Switch3/1 -> LcACC_TiRemChanged_flg/1

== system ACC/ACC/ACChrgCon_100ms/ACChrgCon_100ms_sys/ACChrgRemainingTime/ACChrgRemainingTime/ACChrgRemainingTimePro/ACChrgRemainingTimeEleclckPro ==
  LcACC_ChrgingTiRem_min : Inport
  GeODP_ObcElecLck_enum : Inport  Port=2
  LcACC_TiRemPro_min : Inport  Port=3
  BMSDelay1 : AIWAYS_Powertrain_BMS_lib/Debounce & Delay/BMSDelay
  Constant11 : Constant  Value=Enum_ODPElockState.Enum_ODPElockState_UnLock
  Constant3 : Constant  Value=ASWTYPE_TRUE
  Constant6 : Constant  Value=ASWTYPE_FALSE
  Constant7 : Constant  Value=CcACC_Initial700Ti_ms
  Constant8 : Constant  Value=ACC_RUNTIME_MS
  Data Type Conversion3 : DataTypeConversion
  EdgeRising : AIWAYS_Powertrain_BMS_lib/Logical Operators/EdgeRising
  Relational Operator4 : RelationalOperator  Operator===  OutDataTypeStr=boolean
  Relational Operator5 : RelationalOperator  Operator===  OutDataTypeStr=boolean
  StateRetention : Subsystem
  Switch1 : Switch  Criteria=u2 ~= 0
  Switch3 : Switch  Criteria=u2 ~= 0
  LcACC_TiRemEleclckPro_min : Outport
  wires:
  Constant3/1 -> BMSDelay1/1
  BMSDelay1/1 -> Relational Operator5/1
  Relational Operator5/1 -> Switch3/2
  Constant6/1 -> Relational Operator5/2
  Constant8/1 -> BMSDelay1/2
  Constant7/1 -> BMSDelay1/3
  GeODP_ObcElecLck_enum/1 -> Data Type Conversion3/1
  Data Type Conversion3/1 -> Relational Operator4/1
  Constant11/1 -> Relational Operator4/2
  Relational Operator4/1 -> EdgeRising/1, Switch3/1
  EdgeRising/1 -> Switch3/3
  Switch3/1 -> StateRetention/1(set)
  StateRetention/1(LbACC_ElecLckUnlock_flg) -> Switch1/2
  LcACC_TiRemPro_min/1 -> Switch1/3
  LcACC_ChrgingTiRem_min/1 -> Switch1/1
  Switch1/1 -> LcACC_TiRemEleclckPro_min/1

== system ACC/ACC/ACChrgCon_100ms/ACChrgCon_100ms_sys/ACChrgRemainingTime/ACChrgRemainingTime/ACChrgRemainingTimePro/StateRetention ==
  set : Inport
  Constant3 : Constant  Value=ACC_CONST0_NUMB
  Constant4 : Constant  Value=CcACC_RemTimeHold_ms
  Constant5 : Constant  Value=ACC_RUNTIME_MS
  Data Type Conversion1 : DataTypeConversion  OutDataTypeStr=single
  Data Type Conversion2 : DataTypeConversion  OutDataTypeStr=single
  EdgeRising : AIWAYS_Powertrain_BMS_lib/Logical Operators/EdgeRising
  Relational Operator3 : RelationalOperator  Operator=>  OutDataTypeStr=boolean
  Subsystem : Subsystem
  Subsystem1 : Subsystem
  Unit Delay1 : UnitDelay  SampleTime=-1  StateName=StateName
  LcACC_TiRemEq_flg : Outport
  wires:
  Subsystem1/1(Timer) -> Relational Operator3/1
  Relational Operator3/1 -> Unit Delay1/1
  Constant5/1 -> Data Type Conversion2/1
  Constant3/1 -> Data Type Conversion1/1
  set/1 -> Subsystem/1(set)
  Constant4/1 -> Relational Operator3/2
  Subsystem/1(Q) -> LcACC_TiRemEq_flg/1, Subsystem1/1(En)
  EdgeRising/1 -> Subsystem1/3(Rst)
  Unit Delay1/1 -> EdgeRising/1, Subsystem/2(clear)
  Data Type Conversion1/1 -> Subsystem1/4(Vst)
  Data Type Conversion2/1 -> Subsystem1/2(Ts)

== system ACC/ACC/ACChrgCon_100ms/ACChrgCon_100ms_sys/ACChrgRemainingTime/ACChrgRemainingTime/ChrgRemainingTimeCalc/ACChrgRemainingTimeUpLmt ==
  note: 2000
  GcODP_MaxPwrObcChrg_W : Inport
  Constant1 : Constant  Value=CcACC_ChrgPwr3_W
  Constant13 : Constant  Value=CcACC_RemTimeHighThrhd3_min
  Constant15 : Constant  Value=CcACC_ChrgPwr1_W
  Constant16 : Constant  Value=CcACC_RemTimeHighThrhd1_min
  Constant17 : Constant  Value=CcACC_ChrgPwr2_W
  Constant18 : Constant  Value=CcACC_RemTimeHighThrhd2_min
  Constant19 : Constant  Value=CcACC_ChrgPwr1_W
  Constant2 : Constant  Value=CcACC_ChrgPwr3_W
  Constant3 : Constant  Value=CcACC_RemTimeHighThrhd4_min
  Data Type Conversion1 : DataTypeConversion
  Logical Operator1 : Logic  AllPortsSameDT=off  OutDataTypeStr=boolean
  Logical Operator2 : Logic  AllPortsSameDT=off  OutDataTypeStr=boolean
  Relational Operator1 : RelationalOperator  Operator=<=  OutDataTypeStr=boolean
  Relational Operator2 : RelationalOperator  OutDataTypeStr=boolean
  Relational Operator3 : RelationalOperator  Operator=<=  OutDataTypeStr=boolean
  Relational Operator4 : RelationalOperator  Operator=>  OutDataTypeStr=boolean
  Relational Operator5 : RelationalOperator  Operator=>  OutDataTypeStr=boolean
  Switch1 : Switch  Criteria=u2 ~= 0
  Switch5 : Switch  Criteria=u2 ~= 0
  Switch6 : Switch  Criteria=u2 ~= 0
  LcACC_RemainingTimeUpLmt_min : Outport
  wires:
  Relational Operator4/1 -> Logical Operator2/2
  Constant16/1 -> Switch5/1
  Constant15/1 -> Relational Operator4/2
  Constant17/1 -> Relational Operator2/2
  Constant13/1 -> Switch6/3
  Data Type Conversion1/1 -> Relational Operator5/1, Relational Operator3/1, Relational Operator2/1, Relational Operator4/1, Relational Operator1/1
  Relational Operator2/1 -> Logical Operator1/1
  Constant18/1 -> Switch6/1
  Switch6/1 -> Switch5/3
  Constant19/1 -> Relational Operator3/2
  GcODP_MaxPwrObcChrg_W/1 -> Data Type Conversion1/1
  Relational Operator3/1 -> Logical Operator1/2
  Switch1/1 -> LcACC_RemainingTimeUpLmt_min/1
  Logical Operator1/1 -> Switch6/2
  Logical Operator2/1 -> Switch5/2
  Constant1/1 -> Relational Operator1/2
  Relational Operator1/1 -> Logical Operator2/1
  Switch5/1 -> Switch1/3
  Relational Operator5/1 -> Switch1/2
  Constant2/1 -> Relational Operator5/2
  Constant3/1 -> Switch1/1

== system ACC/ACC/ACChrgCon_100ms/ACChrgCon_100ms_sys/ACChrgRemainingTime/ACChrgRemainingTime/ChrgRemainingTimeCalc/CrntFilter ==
  GcHDP_PackCrnt_A : Inport
  LcACC_FilterCrnt1_A : Inport  Port=2
  GcHDP_PackVolt_V : Inport  Port=3
  GcODP_ObcCpDuty_numb : Inport  Port=4
  GeODP_ObcElecLck_enum : Inport  Port=5
  GcVDP_ChrgLdReq_numb : Inport  Port=6
  GeODP_ObcCcSt_enum : Inport  Port=7
  Abs : Abs
  BMSDelay : AIWAYS_Powertrain_BMS_lib/Debounce & Delay/BMSDelay
  Constant : Constant  Value=ASWTYPE_TRUE
  Constant20 : Constant  Value=ASWTYPE_FALSE
  Constant4 : Constant  Value=CcACC_CrntFilterTi2_ms
  Constant5 : Constant  Value=ACC_RUNTIME_MS
  CrntTransform : Subsystem
  Moving Average : Subsystem  TreatAsAtomicUnit=on  mask(MovingAverage00){BufferSize=CcACC_CrntFilterTi2_cnt}
      mask prompts: BufferSize "Buffer size"
      mask help: Block will compute the moving average of the input signal based on the number of samples input as the buffer_size. NOTE: Will not work with vectorized inputs. Default buffer size = 2. Input1=Value; Input2=Reset
  OBCElecLckUnlock : Subsystem
  Product4 : Product  OutDataTypeStr=Inherit: Inherit via back propagation
  Switch1 : Switch  Criteria=u2 ~= 0
  Switch2 : Switch  Criteria=u2 ~= 0
  LcACC_FilterPwr_W : Outport
  LcACC_FilterCrnt_A : Outport  Port=2
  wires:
  BMSDelay/1 -> Switch1/2
  Switch1/1 -> LcACC_FilterCrnt_A/1, Product4/2
  Constant20/1 -> Moving Average/2(R)
  GcHDP_PackCrnt_A/1 -> CrntTransform/1(GcHDP_PackCrnt_A), Moving Average/1(u)
  Constant4/1 -> BMSDelay/3
  Constant/1 -> BMSDelay/1
  GcHDP_PackVolt_V/1 -> Product4/1, CrntTransform/3(GcHDP_PackVolt_V)
  Constant5/1 -> BMSDelay/2
  Moving Average/1(y) -> Switch1/1
  Abs/1 -> LcACC_FilterPwr_W/1
  Product4/1 -> Abs/1
  LcACC_FilterCrnt1_A/1 -> Switch2/3
  GeODP_ObcElecLck_enum/1 -> OBCElecLckUnlock/2(GeODP_ObcElecLck_enum)
  GeODP_ObcCcSt_enum/1 -> OBCElecLckUnlock/3(GeODP_ObcCcSt_enum)
  OBCElecLckUnlock/1(LbACC_ElecLckUnlock_flg) -> Switch2/2
  GcODP_ObcCpDuty_numb/1 -> CrntTransform/4(GcODP_ObcCpDuty_numb), OBCElecLckUnlock/1(GcODP_ObcCpDuty_numb)
  CrntTransform/1(LcACC_TrsformCrnt_A) -> Switch2/1
  Switch2/1 -> Switch1/3
  GcVDP_ChrgLdReq_numb/1 -> CrntTransform/2(GcVDP_ChrgLdReq_numb)

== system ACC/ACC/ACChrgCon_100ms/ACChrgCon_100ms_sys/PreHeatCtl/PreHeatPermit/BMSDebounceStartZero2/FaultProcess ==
  Signal : Inport
  Hearl2Fault : Inport  Port=2
  FaultStep : Inport  Port=3
  FaultFlagOldState : Inport  Port=4
  Constant : Constant  OutDataTypeStr=Inherit: Inherit via back propagation
  Constant1 : Constant  Value=0  OutDataTypeStr=Inherit: Inherit via back propagation
  Decrease : Subsystem
  Increase : Subsystem
  Relational Operator : RelationalOperator  OutDataTypeStr=boolean
  Switch : Switch  Criteria=u2 ~= 0
  Switch1 : Switch  Criteria=u2 ~= 0
  Switch2 : Switch  Criteria=u2 ~= 0
  Unit Delay : UnitDelay  SampleTime=-1  StateName=StateName
  Unit Delay1 : UnitDelay  SampleTime=-1  StateName=StateName
  FaultFlag : Outport
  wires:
  Unit Delay1/1 -> Switch2/2
  Unit Delay/1 -> Switch2/3
  Switch2/1 -> Increase/2(Counter), Decrease/2(Counter)
  Constant1/1 -> Switch2/1
  Constant/1 -> Switch/1
  FaultFlagOldState/1 -> Switch/3
  Switch/1 -> FaultFlag/1
  Relational Operator/1 -> Switch/2, Unit Delay1/1
  FaultStep/1 -> Increase/1(FaultStep), Decrease/1(FaultStep)
  Hearl2Fault/1 -> Relational Operator/2
  Switch1/1 -> Relational Operator/1, Unit Delay/1
  Decrease/1(FaultCnt) -> Switch1/3
  Increase/1(FaultCnt) -> Switch1/1
  Signal/1 -> Switch1/2

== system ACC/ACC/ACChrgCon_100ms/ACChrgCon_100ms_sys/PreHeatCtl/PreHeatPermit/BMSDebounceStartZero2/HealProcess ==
  Signal : Inport
  Fault2Heal : Inport  Port=2
  HealStep : Inport  Port=3
  FaultFlagOldState : Inport  Port=4
  Compare To Zero : simulink/Logic and Bit Operations/Compare To Zero  relop===  OutDataTypeStr=boolean
  Constant : Constant  Value=0  OutDataTypeStr=Inherit: Inherit via back propagation
  Constant1 : Constant  Value=0  OutDataTypeStr=Inherit: Inherit via back propagation
  Decrease : Subsystem
  Increase : Subsystem
  Relational Operator : RelationalOperator  OutDataTypeStr=boolean
  Switch : Switch  Criteria=u2 ~= 0
  Switch1 : Switch  Criteria=u2 ~= 0
  Switch2 : Switch  Criteria=u2 ~= 0
  Unit Delay1 : UnitDelay  SampleTime=-1  StateName=StateName
  Unit Delay2 : UnitDelay  SampleTime=-1  StateName=StateName
  FaultFlag : Outport
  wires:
  Switch2/1 -> Decrease/2(Counter), Increase/2(Counter)
  Unit Delay2/1 -> Switch2/2
  Unit Delay1/1 -> Switch2/3
  Constant1/1 -> Switch2/1
  Compare To Zero/1 -> Switch1/2
  Constant/1 -> Switch/1
  FaultFlagOldState/1 -> Switch/3
  Switch/1 -> FaultFlag/1
  Relational Operator/1 -> Switch/2, Unit Delay2/1
  Signal/1 -> Compare To Zero/1
  Increase/1(HealCnt) -> Switch1/1
  Decrease/1(HealCnt) -> Switch1/3
  Switch1/1 -> Relational Operator/1, Unit Delay1/1
  Fault2Heal/1 -> Relational Operator/2
  HealStep/1 -> Increase/1(HealStep), Decrease/1(HealStep)

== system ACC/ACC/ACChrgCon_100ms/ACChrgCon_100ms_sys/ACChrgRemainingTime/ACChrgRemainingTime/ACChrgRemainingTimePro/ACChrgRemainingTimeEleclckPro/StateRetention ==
  set : Inport
  Constant : Constant  Value=ASWTYPE_TRUE
  Constant3 : Constant  Value=ACC_CONST0_NUMB
  Constant4 : Constant  Value=CcACC_ElecLckRemTimeHold_ms
  Constant5 : Constant  Value=ACC_RUNTIME_MS
  Data Type Conversion1 : DataTypeConversion  OutDataTypeStr=single
  Data Type Conversion2 : DataTypeConversion  OutDataTypeStr=single
  EdgeRising : AIWAYS_Powertrain_BMS_lib/Logical Operators/EdgeRising
  Logical Operator2 : Logic  Operator=OR  AllPortsSameDT=off  OutDataTypeStr=boolean
  Relational Operator3 : RelationalOperator  Operator=>  OutDataTypeStr=boolean
  Relational Operator5 : RelationalOperator  Operator===  OutDataTypeStr=boolean
  Subsystem : Subsystem
  Subsystem1 : Subsystem
  Unit Delay1 : UnitDelay  SampleTime=-1  StateName=StateName
  LbACC_ElecLckUnlock_flg : Outport
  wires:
  Subsystem1/1(Timer) -> Relational Operator3/1
  Relational Operator3/1 -> Unit Delay1/1
  Constant5/1 -> Data Type Conversion2/1
  Constant3/1 -> Data Type Conversion1/1
  set/1 -> Relational Operator5/1, Subsystem/2(set)
  Constant4/1 -> Relational Operator3/2
  Subsystem/1(Q) -> LbACC_ElecLckUnlock_flg/1, Subsystem1/1(En)
  EdgeRising/1 -> Logical Operator2/2
  Unit Delay1/1 -> Subsystem/1(clear), EdgeRising/1
  Constant/1 -> Relational Operator5/2
  Relational Operator5/1 -> Logical Operator2/1
  Logical Operator2/1 -> Subsystem1/3(Rst)
  Data Type Conversion1/1 -> Subsystem1/4(Vst)
  Data Type Conversion2/1 -> Subsystem1/2(Ts)

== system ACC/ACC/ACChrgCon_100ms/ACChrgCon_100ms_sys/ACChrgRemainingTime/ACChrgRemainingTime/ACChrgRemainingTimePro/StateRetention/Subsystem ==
  set : Inport
  clear : Inport  Port=2
  Logical Operator1 : Logic  AllPortsSameDT=off  OutDataTypeStr=boolean
  Logical Operator2 : Logic  Operator=OR  AllPortsSameDT=off  OutDataTypeStr=boolean
  Logical2 : Logic  Operator=NOT  OutDataTypeStr=boolean
  Unit Delay1 : UnitDelay  SampleTime=-1  StateName=StateName
  Q : Outport
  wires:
  set/1 -> Logical Operator2/2
  Logical Operator1/1 -> Q/1, Unit Delay1/1
  Logical Operator2/1 -> Logical Operator1/1
  clear/1 -> Logical2/1
  Unit Delay1/1 -> Logical Operator2/1
  Logical2/1 -> Logical Operator1/2

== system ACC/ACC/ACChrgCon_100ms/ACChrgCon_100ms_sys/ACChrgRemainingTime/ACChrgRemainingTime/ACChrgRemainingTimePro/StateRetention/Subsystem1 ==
  En : Inport
  Ts : Inport  Port=2
  Rst : Inport  Port=3
  Vst : Inport  Port=4
  Constant2 : Constant  Value=ACC_CONST0_NUMB
  Data Type Conversion1 : DataTypeConversion
  Sum2 : Sum  OutDataTypeStr=Inherit: Inherit via back propagation  RndMeth=Zero
  Switch1 : Switch  Criteria=u2 ~= 0
  Switch2 : Switch  Criteria=u2 ~= 0
  Unit Delay1 : UnitDelay  SampleTime=-1  StateName=StateName
  Timer : Outport
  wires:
  Vst/1 -> Switch1/1
  Rst/1 -> Switch1/2
  Ts/1 -> Switch2/1
  En/1 -> Switch2/2
  Switch2/1 -> Sum2/1
  Unit Delay1/1 -> Sum2/2
  Sum2/1 -> Switch1/3
  Switch1/1 -> Unit Delay1/1, Timer/1
  Constant2/1 -> Data Type Conversion1/1
  Data Type Conversion1/1 -> Switch2/3

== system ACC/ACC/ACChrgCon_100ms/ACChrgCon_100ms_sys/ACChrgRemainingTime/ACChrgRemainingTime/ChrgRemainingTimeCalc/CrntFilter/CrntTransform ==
  GcHDP_PackCrnt_A : Inport
  GcVDP_ChrgLdReq_numb : Inport  Port=2
  GcHDP_PackVolt_V : Inport  Port=3
  GcODP_ObcCpDuty_numb : Inport  Port=4
  Constant12 : Constant  Value=ACC_CONST1000_NUMB
  Constant4 : Constant  Value=ACC_CONST121_NUMB
  Constant5 : Constant  Value=CcACC_OBCChrgPwr_W
  Product1 : Product  OutDataTypeStr=Inherit: Inherit via back propagation
  Product2 : Product  Inputs=**/  OutDataTypeStr=Inherit: Inherit via back propagation
  Product4 : Product  OutDataTypeStr=Inherit: Inherit via back propagation
  Product6 : Product  Inputs=*/  OutDataTypeStr=Inherit: Inherit via back propagation
  Sum1 : Sum  OutDataTypeStr=Inherit: Inherit via back propagation  RndMeth=Zero
  Sum2 : Sum  Inputs=+-  OutDataTypeStr=Inherit: Inherit via back propagation  RndMeth=Zero
  LcACC_TrsformCrnt_A : Outport
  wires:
  GcODP_ObcCpDuty_numb/1 -> Product4/1
  Constant4/1 -> Product4/2
  Product4/1 -> Product6/1
  Constant5/1 -> Product6/2
  Product6/1 -> Product1/1
  Sum1/1 -> Product1/2
  GcVDP_ChrgLdReq_numb/1 -> Product2/1
  GcHDP_PackVolt_V/1 -> Product2/3
  Product2/1 -> Sum2/2, Sum1/2
  GcHDP_PackCrnt_A/1 -> Sum1/1
  Product1/1 -> Sum2/1
  Sum2/1 -> LcACC_TrsformCrnt_A/1
  Constant12/1 -> Product2/2

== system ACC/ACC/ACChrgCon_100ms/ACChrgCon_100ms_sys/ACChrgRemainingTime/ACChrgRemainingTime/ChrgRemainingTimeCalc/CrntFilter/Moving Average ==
  note: Moving Average
  u : Inport
  R : Inport  Port=2  OutDataTypeStr=boolean
  Chart : Stateflow chart  TreatAsAtomicUnit=on
  Signal Conversion : SignalConversion  ConversionOutput=Contiguous copy  OverrideOpt=off
  y : Outport
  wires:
  Signal Conversion/1 -> y/1
  Chart/1(Y) -> Signal Conversion/1
  u/1 -> Chart/1(u)
  R/1 -> Chart/2(R)

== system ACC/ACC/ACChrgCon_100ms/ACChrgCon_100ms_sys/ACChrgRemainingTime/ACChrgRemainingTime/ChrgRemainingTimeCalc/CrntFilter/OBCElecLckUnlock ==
  GcODP_ObcCpDuty_numb : Inport
  GeODP_ObcElecLck_enum : Inport  Port=2
  GeODP_ObcCcSt_enum : Inport  Port=3
  BMSDelay1 : AIWAYS_Powertrain_BMS_lib/Debounce & Delay/BMSDelay
  Constant1 : Constant  Value=ASWTYPE_TRUE
  Constant11 : Constant  Value=Enum_ODPElockState.Enum_ODPElockState_UnLock
  Constant14 : Constant  Value=Enum_ODPCCState.Enum_ODPCCState_ChrgConnect32A220
  Constant2 : Constant  Value=ASWTYPE_FALSE
  Constant3 : Constant  Value=CcACC_Initial700Ti_ms
  Constant6 : Constant  Value=ACC_RUNTIME_MS
  Constant7 : Constant  Value=CcACC_CPDutyLowThrhd_pct
  Data Type Conversion2 : DataTypeConversion
  Data Type Conversion3 : DataTypeConversion
  Logical Operator : Logic  Inputs=4  AllPortsSameDT=off  OutDataTypeStr=boolean
  Relational Operator10 : RelationalOperator  Operator===  OutDataTypeStr=boolean
  Relational Operator2 : RelationalOperator  Operator=>  OutDataTypeStr=boolean
  Relational Operator3 : RelationalOperator  Operator===  OutDataTypeStr=boolean
  Relational Operator4 : RelationalOperator  Operator===  OutDataTypeStr=boolean
  LbACC_ElecLckUnlock_flg : Outport
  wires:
  Logical Operator/1 -> LbACC_ElecLckUnlock_flg/1
  Relational Operator10/1 -> Logical Operator/1
  Relational Operator3/1 -> Logical Operator/3
  Constant1/1 -> BMSDelay1/1
  Constant2/1 -> Relational Operator3/2
  Constant7/1 -> Relational Operator2/2
  Relational Operator2/1 -> Logical Operator/2
  BMSDelay1/1 -> Relational Operator3/1
  GcODP_ObcCpDuty_numb/1 -> Relational Operator2/1
  Relational Operator4/1 -> Logical Operator/4
  Constant11/1 -> Relational Operator4/2
  Data Type Conversion3/1 -> Relational Operator4/1
  Constant14/1 -> Relational Operator10/2
  GeODP_ObcCcSt_enum/1 -> Data Type Conversion2/1
  Constant6/1 -> BMSDelay1/2
  Constant3/1 -> BMSDelay1/3
  Data Type Conversion2/1 -> Relational Operator10/1
  GeODP_ObcElecLck_enum/1 -> Data Type Conversion3/1

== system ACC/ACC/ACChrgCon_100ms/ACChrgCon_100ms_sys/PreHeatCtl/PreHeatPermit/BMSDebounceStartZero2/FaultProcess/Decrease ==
  FaultStep : Inport
  Counter : Inport  Port=2
  Constant : Constant  Value=0  OutDataTypeStr=Inherit: Inherit via back propagation
  Nomal : Subsystem
  Relational Operator : RelationalOperator  OutDataTypeStr=boolean
  Switch : Switch  Criteria=u2 ~= 0
  FaultCnt : Outport
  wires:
  Constant/1 -> Switch/3
  FaultStep/1 -> Relational Operator/2, Nomal/1(FaultStep)
  Counter/1 -> Relational Operator/1, Nomal/2(Counter)
  Switch/1 -> FaultCnt/1
  Nomal/1(FaultCnt) -> Switch/1
  Relational Operator/1 -> Switch/2
